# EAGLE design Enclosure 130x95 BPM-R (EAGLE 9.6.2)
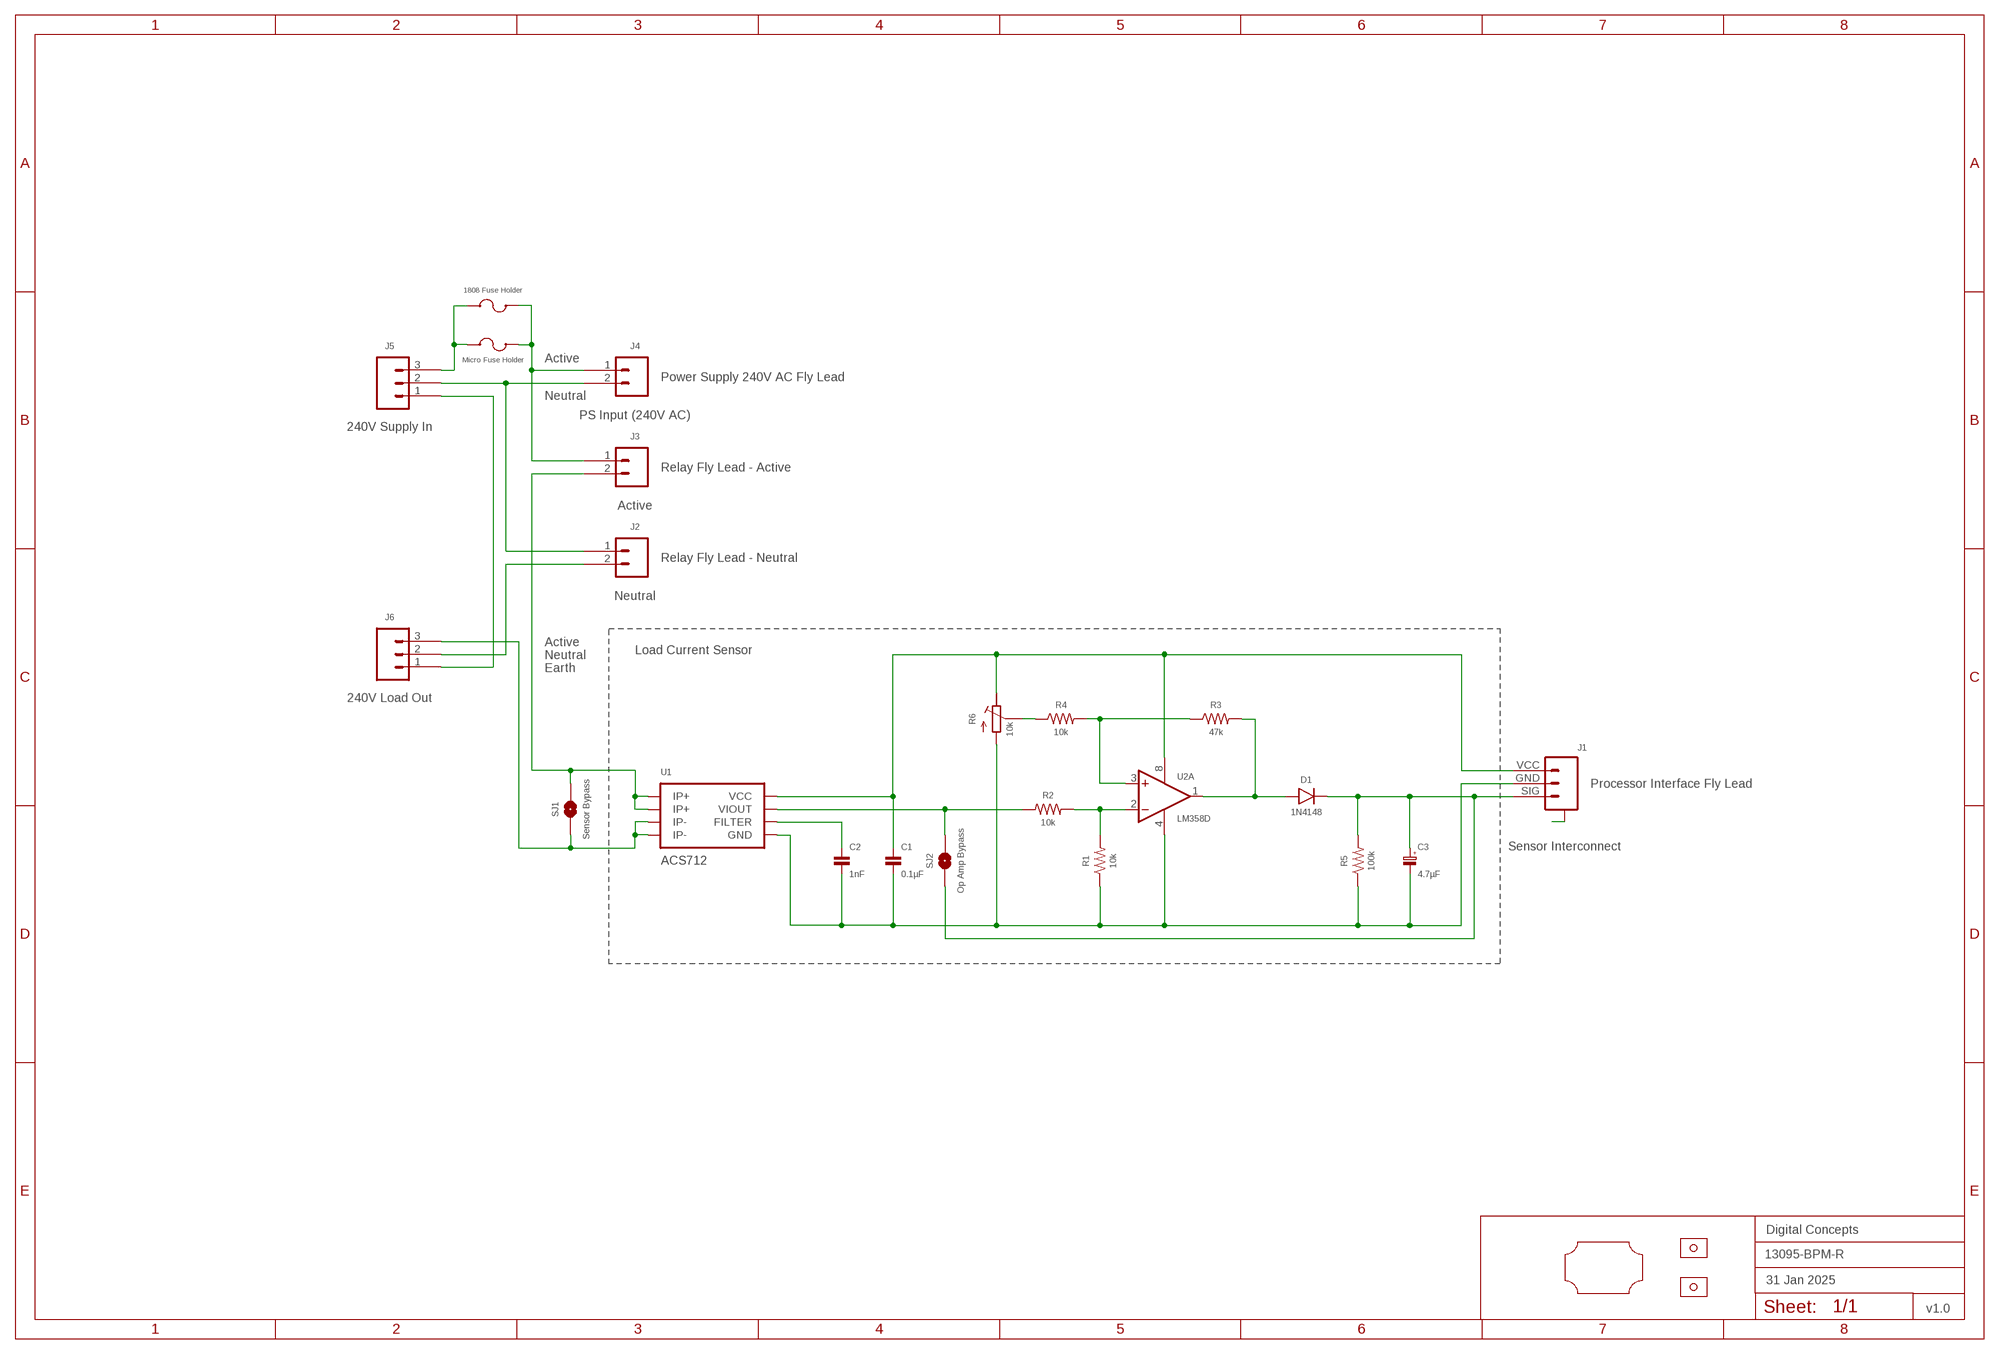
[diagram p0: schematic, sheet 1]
FRAME2 (A3L-LOC): DATE: 31 Jan 2025; OWNER: Digital Concepts; TITLE: 13095-BPM-R; VERSION: v1.0

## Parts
C1  0.1µF  CAPACITOR-0805  [C0805]
C2  1nF  CAPACITOR-0805  [C0805]
C3  4.7µF  CAPACITOR-1206-TANTALUM  [C1206-POLARISED]
D1  1N4148  DIODE-1N4148-SOD323  [SOD-323]
F2  1808 Fuse Holder  FUSE-HOLDER-1808  [FUSE-HOLDER-1808]
J1  Sensor Interconnect  JST-SH1.0-3-SMD-HORIZONTAL-SIG  [JST-SH1.0-3-HORIZONTAL-SIG]
J2  Neutral  TERMINAL_SCREW_2P_VERTICAL  [TERMINAL-SCREW-2P]
J3  Active  TERMINAL_SCREW_2P_VERTICAL  [TERMINAL-SCREW-2P]
J4  PS Input (240V AC)  JST-XH2.54-2-HORIZONTAL  [JST-XH2.4-2-HORIZONTAL]
J5  240V Supply In  TERMINAL_SCREW_3P_VERTICAL  [TERMINAL-SCREW-3P]
J6  240V Load Out  TERMINAL_SCREW_3P_VERTICAL  [TERMINAL-SCREW-3P]
R1  10k  RESISTORR0805  [R0805]
R2  10k  RESISTORR0805  [R0805]
R3  47k  RESISTORR0805  [R0805]
R4  10k  RESISTORR0805  [R0805]
R5  100k  RESISTORR0805  [R0805]
R6  10k  RESISTOR-TRIMM-3386P  [RTRIM3386P]
SJ1  Sensor Bypass  SJ  [SJ]
SJ2  Op Amp Bypass  SJ  [SJ]
U1  ACS712  [SOP-8]
U2  LM358D  [SOP-8]
U$1  PCB-OUTLINE-130X95-MAX-RC-H3  [PROTO-130X95-OUTLINE-MAX-RC-H3]
U$2  Micro Fuse Holder  FUSE-HOLDER  [FUSE-HOLDER-MICRO]
U$4  STRAIN-RELIEF-SADDLE  [STRAIN-RELIEF-SADDLE]
U$5  STRAIN-RELIEF-SADDLE  [STRAIN-RELIEF-SADDLE]

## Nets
A: J1.A@1(A) J1.A@3(A)
ACTIVE_IN: F2.P$2 J3.1 J4.1 U$2.P$3 U$2.P$4
ACTIVE_OUT: J3.2 SJ1.2 U1.1(IP+) U1.2(IP+)
EARTH: J5.1 J6.1
N$2: C1.1 J1.VCC R6.1(E) U1.8(VCC) U2.8(P:V+)
N$3: C3.1(+) D1.C J1.SIG R5.2 SJ2.1
N$4: D1.A R3.2 U2.1(A:OUT)
N$5: R3.1 R4.2 U2.3(A:+IN)
N$6: R4.1 R6.2(S)
N$7: F2.P$1 J5.3 U$2.P$1 U$2.P$2
N$8: R1.2 R2.2 U2.2(A:-IN)
N$19: J6.3 SJ1.1 U1.3(IP-) U1.4(IP-)
N$20: C1.2 C2.2 C3.2(-) J1.GND R1.1 R5.1 R6.3(A) U1.5(GND) U2.4(P:V-)
N$22: R2.1 SJ2.2 U1.7(VIOUT)
N$24: C2.1 U1.6(FILTER)
NEUTRAL_IN: J2.1 J4.2 J5.2
NEUTRAL_OUT: J2.2 J6.2
Unconnected: U2.5(B:+IN) U2.6(B:-IN) U2.7(B:OUT)

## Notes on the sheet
- Active
- Power Supply 240V AC Fly Lead
- Neutral
- Relay Fly Lead - Active
- Relay Fly Lead - Neutral
- Active
- Neutral | Load Current Sensor
- Earth
- Processor Interface Fly Lead

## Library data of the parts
C1 C2 = digitalconcepts:CAPACITOR-0805: 0805 Capacitor
C3 = digitalconcepts:CAPACITOR-1206-TANTALUM: Capacitor 1206 Tantalum
D1 = digitalconcepts:DIODE-1N4148-SOD323: 1N4148 SOD-323
F2 = digitalconcepts:FUSE-HOLDER-1808: 1808 Fuse Holder
J1 = digitalconcepts:JST-SH1.0-3-SMD-HORIZONTAL-SIG: JST SH1.0 3P SMD Horizontal Connector with Signal
J2 J3 = digitalconcepts:TERMINAL_SCREW_2P_VERTICAL: PCB Mount Screw-Type Terminal 2P
J4 = digitalconcepts:JST-XH2.54-2-HORIZONTAL: XH2.54 2P Horizontal Connector
J5 J6 = digitalconcepts:TERMINAL_SCREW_3P_VERTICAL: PCB Mount Screw-Type Terminal 3P
R1-R5 = digitalconcepts:RESISTOR: Resistor; SPICEPREFIX: R
R6 = digitalconcepts:RESISTOR-TRIMM-3386P: BOURNS Trim Pot 3386P
SJ1 SJ2 = digitalconcepts:SJ: Solder Jumper
U1 = digitalconcepts:ACS712: ACS712 Hall-Effect-Based Linear Current Sensor IC
U2 = digitalconcepts:LM358: OP AMP also LM158; LM258; LM2904 Source: http://cache.national.com/ds/LM/LM158.pdf
U$1 = digitalconcepts:PCB-OUTLINE-130X95-MAX-RC-H3: PCB Eagle Max-Right-Cropped outline for 130 x 95 enclosure (Horizontal format)
U$2 = digitalconcepts:FUSE-HOLDER: Fuse Holder
U$4 U$5 = digitalconcepts:STRAIN-RELIEF-SADDLE: Strain Relief Saddle (7mm x 13mm)

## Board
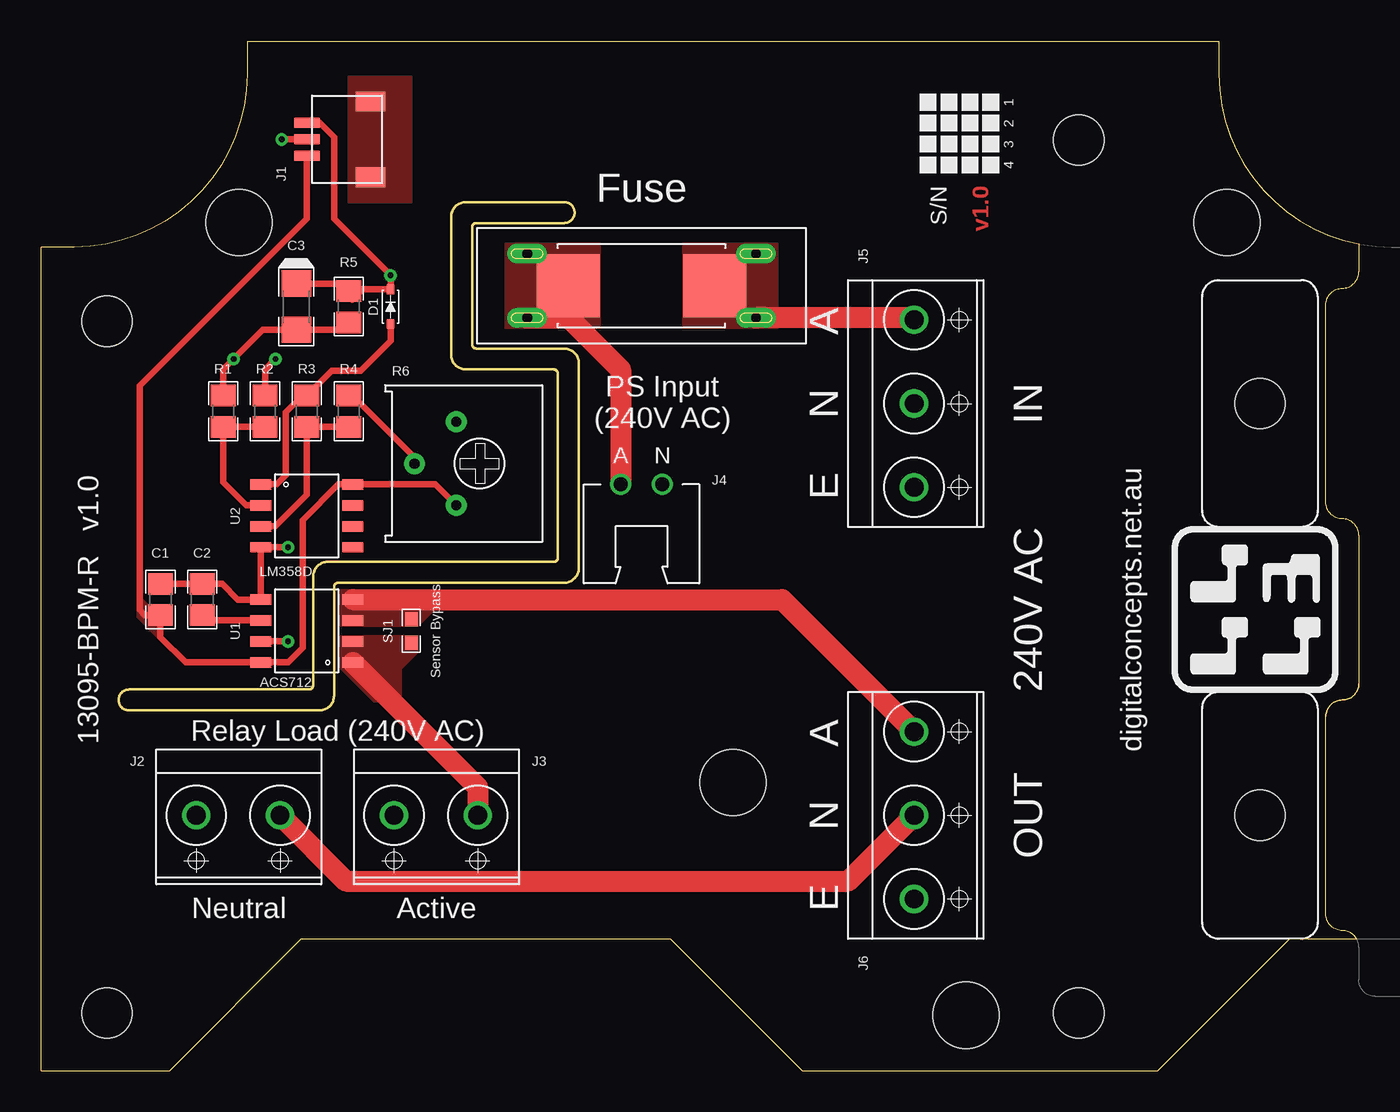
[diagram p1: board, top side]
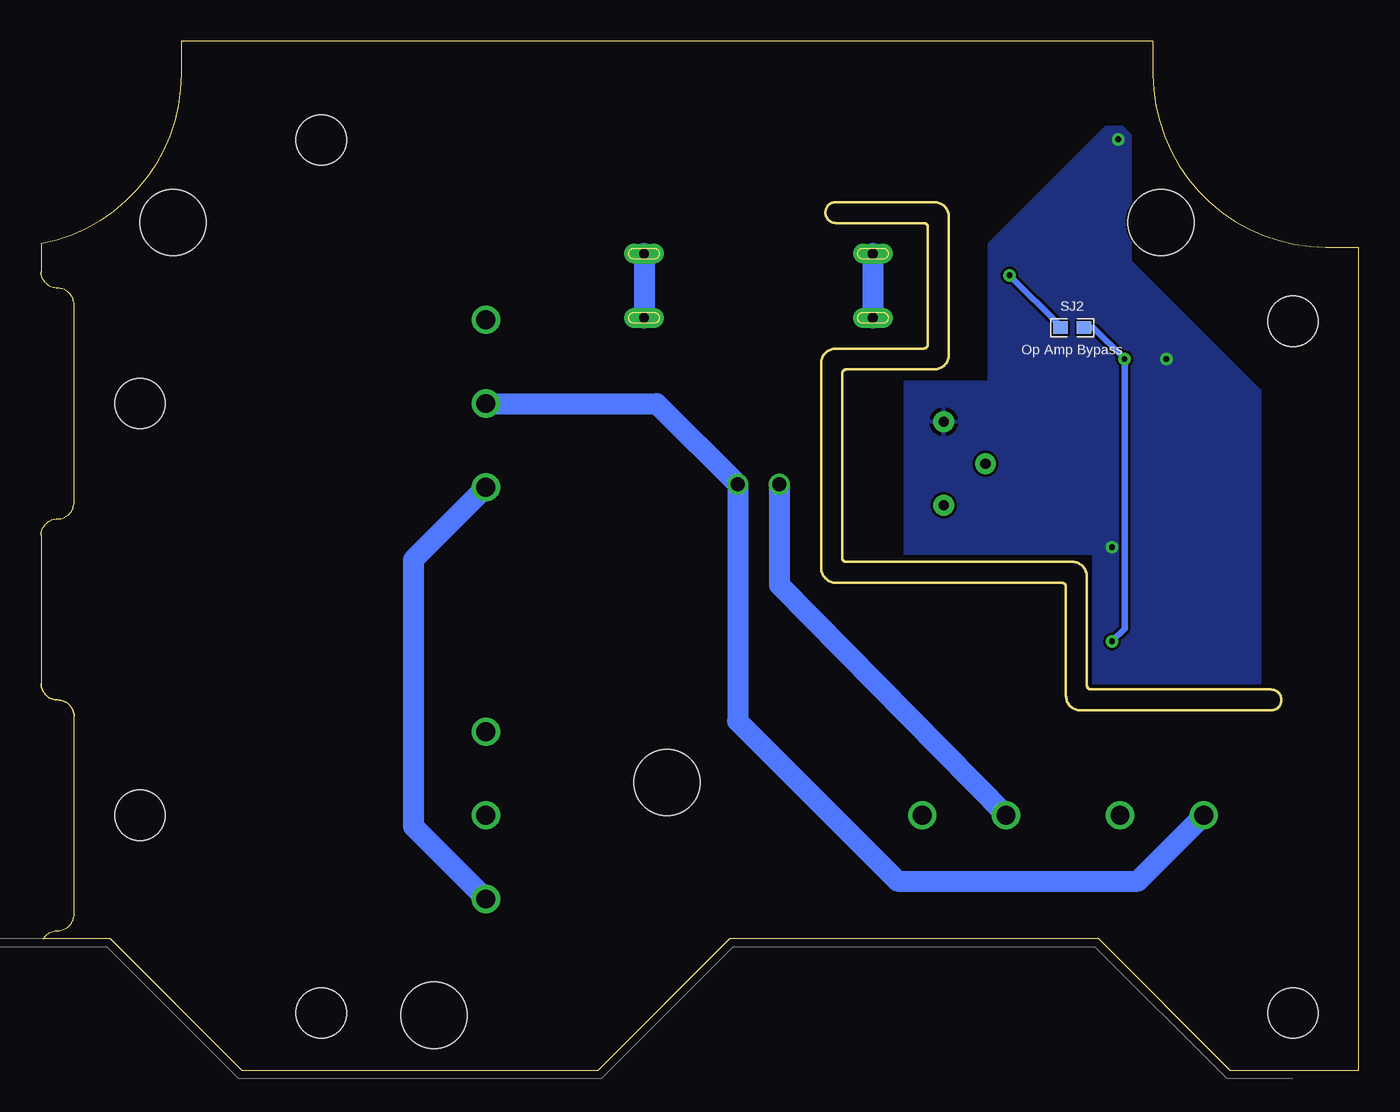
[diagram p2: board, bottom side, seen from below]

Size 80 x 62.5 mm. Coordinates in mm from the lower left corner, seen from the top.
Copper layers (1*16): Top 0.035mm / dielectric 1.5mm / Bottom 0.035mm
Design rules "default *": minimum track width 6mil, minimum drill 0.35mm, track to track 6mil, track to pad 6mil, pad to pad 6mil, via to via 6mil, smd to smd 6mil, copper to edge 6mil, drill to drill 6mil, minimum pad ring 1mil, minimum via ring 8mil, stop-mask expansion 4mil, vias tented up to drill 0mil, thermal gap 10mil
Milling: 28 lines

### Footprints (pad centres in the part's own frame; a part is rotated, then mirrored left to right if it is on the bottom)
C0805 = smd 1.3 x 1.5: 1 -0.95,0; 2 0.95,0
C1206-POLARISED = smd 1.6 x 1.8: 1 -1.4,0; 2 1.4,0
SOD-323 = smd 0.59 x 0.45: A -1.055,0; C 1.055,0
FUSE-HOLDER-1808 = smd 3.81 x 3.81: P$1 -4.445,0; P$2 4.445,0
JST-SH1.0-3-HORIZONTAL-SIG = smd 1.2 x 1.8: A@1 -2.3,-1.335; A@3 2.3,-1.335 | smd 0.6 x 1.55: GND 0,2.54; SIG 1,2.54; VCC -1,2.54
TERMINAL-SCREW-2P = drill 1.143: 1 -2.58,0; 2 2.5,0
JST-XH2.4-2-HORIZONTAL = drill 0.85: 1 1.27,0; 2 -1.27,0
TERMINAL-SCREW-3P = drill 1.143: 1 -5.08,0; 2 0,0; 3 5.08,0
R0805 = smd 1.3 x 1.5: 1 -0.95,0; 2 0.95,0
RTRIM3386P = drill 0.61 pad 1.27: 1 2.54,-0.45; 2 0,-2.99; 3 -2.54,-0.45
SJ = smd 0.864 x 0.762: 1 -0.711,0; 2 0.711,0
SOP-8 = smd 0.635 x 1.27: 1 -1.905,-2.794; 2 -0.635,-2.794; 3 0.635,-2.794; 4 1.905,-2.794; 5 1.905,2.794; 6 0.635,2.794; 7 -0.635,2.794; 8 -1.905,2.794
PROTO-130X95-OUTLINE-MAX-RC-H3 = hole 3.048: -38,10; 21,21; 21,-32; -38,-32 | hole 4: 0,-18; -30,16; 30,16; 14.14,-32.14
FUSE-HOLDER-MICRO = drill 0.6 pad 1.2 long: P$1 -6.95,1.95; P$2 -6.95,-1.95; P$3 6.95,-1.95; P$4 6.95,1.95
STRAIN-RELIEF-SADDLE = hole 3.048: 0,0

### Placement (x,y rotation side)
C1  7.24,28.6 90 top
C2  9.78,28.6 90 top
C3  15.5,46.38 270 top
D1  21.21,46.38 90 top
F2  36.45,47.65 180 top
J1  18.67,56.54 90 top
J2  12,15.5 0 top
J3  24,15.5 0 top
J4  36.45,35.59 180 top
J5  53,40.5 90 top
J6  53,15.5 90 top
R1  11.05,40.03 270 top
R2  13.59,40.03 270 top
R3  16.13,40.03 90 top
R4  18.67,40.03 270 top
R5  18.67,46.38 90 top
R6  25.66,36.85 270 top
SJ1  22.48,26.7 270 top
SJ2  17.4,45.11 0 bottom
U1  16.13,26.7 90 top
U2  16.13,33.68 270 top
U$1  42,35.5 0 top
U$2  36.45,47.65 180 top
U$4  74,40.5 90 top
U$5  74,15.5 90 top

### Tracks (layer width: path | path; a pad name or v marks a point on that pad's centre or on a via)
A
  pour Top (no thermals): 18.67,60.35 22.48,60.35 22.48,52.73 18.67,52.73
ACTIVE_IN
  Top 1.27: U$2.P$4 32.04,45.7 35.18,42.56 J4.1
  Bottom 1.27: J4.1 35.18,29.49 J3.1 | U$2.P$3 U$2.P$4
  pour Top (no thermals): 28.2,50.19 33.91,50.19 33.91,45.11 28.2,45.11
ACTIVE_OUT
  Top 1.27: J3.2 26.5,17.21 U1.1
  pour Top (no thermals): 18.04,26.44 22.86,26.44 22.86,25.36 21.86,24.36 21.86,22.37 20.22,22.37 18.04,24.55
EARTH
  Bottom 1.27: J5.1 57.41,31.02 57.41,14.82 J6.1
N$2
  Top 0.406: R6.1 23.93,35.59 U2.8 18.04,35.59 15.88,33.43 15.88,25.68 14.99,24.79 U1.8 8.76,24.79 7.24,26.31 C1.1 6.29,27.65 5.97,27.97 5.97,41.57 16.13,51.73 J1.VCC
  pour Top (no thermals): 7.24,26.31 7.24,27.97 6.61,27.97 5.97,28.6 5.97,27.58
N$3  (via drill 0.35)
  Top 0.406: C3.1 18.22,47.78 R5.2 18.88,47.12 18.88,46.8 19.52,47.44 D1.C v21.21,48.28 17.78,51.71 17.78,56.67 16.91,57.54 J1.SIG
  Bottom 0.406: SJ2.1 18.11,45.19 v21.21,48.28
N$4
  Top 0.406: U2.1 14.29,35.59 14.86,36.15 14.86,39.96 15.88,40.98 R3.2 17.65,42.5 19.41,42.5 21.21,44.31 D1.A
N$5
  Top 0.406: U2.3 14.23,33.05 16.13,34.95 R3.1 R4.2
N$6
  Top 0.406: R6.2 22.66,37.24 18.92,40.98 R4.1
N$7
  Top 1.27: U$2.P$1 52.88,45.7 J5.3
  Bottom 1.27: U$2.P$2 U$2.P$1
  pour Top (no thermals): 38.99,50.19 44.7,50.19 44.7,45.11 38.99,45.11
N$8
  Top 0.406: U2.2 12.45,34.31 11.05,35.71 R1.2 R2.2
N$19
  Top 1.27: J6.3 44.98,28.6 U1.4
  pour Top (no thermals): 18.04,29.23 23.75,29.23 24.38,28.6 24.38,28.47 22.86,26.95 18.04,26.95
N$20  (via drill 0.35)
  Top 0.406: C1.2 C2.2 10.99,29.55 11.94,28.6 U1.5 13.33,31.58 U2.4 v14.99,31.77 | R5.1 18.22,44.98 C3.2 13.46,44.98 v11.68,43.2 11.05,42.57 R1.1 | J1.GND v14.61,56.54
  pour Bottom: 15.37,57.3 14.35,57.3 13.84,56.79 13.84,49.17 5.97,41.3 5.97,23.52 16.13,23.52 16.13,31.39 27.56,31.39 27.56,41.81 22.48,41.81 22.48,50.19
N$22  (via drill 0.35)
  Top 0.406: v14.23,43.2 13.59,42.57 R2.1 | v14.99,26.06 U1.7
  Bottom 0.406: v14.99,26.06 14.23,26.82 v14.23,43.2 16.13,45.11 SJ2.2
N$24
  Top 0.406: U1.6 10.1,27.33 C2.1
NEUTRAL_IN
  Bottom 1.27: J5.2 42.63,40.5 J4.2 37.72,21.22 28,11.5 13.42,11.5 J2.1
NEUTRAL_OUT
  Top 1.27: J2.2 18.5,11.5 49,11.5 J6.2

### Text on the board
Top: v1.0
tPlace: 1 | 2 | 3 | 4 | S/N | 13095-BPM-R v1.0 | digitalconcepts.net.au
tNames: Fuse | A | N | IN | PS Input / (240V AC) | A | N | E | 240V AC | Relay Load (240V AC) | A | N | OUT | E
